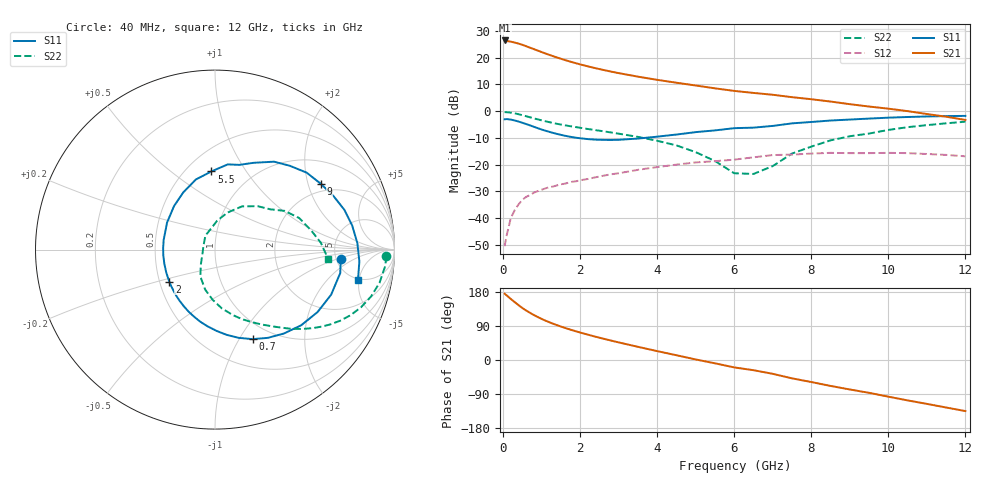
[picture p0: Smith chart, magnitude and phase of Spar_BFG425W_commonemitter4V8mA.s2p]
! Filename: 48bfg425.001
! BFG425W Field C1
! V1=8.298E-001V,V2=4.000E+000V, I1=8.674E-005A, I2=7.990E-003A
# GHz  S  MA  R 50
!  S11  S21  S12  S22
!Freq(GHz)  Mag  Ang  Mag  Ang  Mag  Ang  Mag  Ang
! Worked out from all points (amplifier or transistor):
!   44 points, 40 MHz to 12 GHz, reference 50 ohm
!   highest |S21| = 26.4 dB at 40 MHz (marker M1)
!   |S21| within 3 dB of that: start of sweep to 755.8 MHz
!   unconditionally stable (mu >= 1): 2.059 GHz to end of sweep
!   at 700 MHz: K = 0.48, MSG = 27.5 dB, |S12| = -31.4 dB
!   at 2.4 GHz: K = 1.08, MAG = 18.7 dB, |S12| = -24.7 dB
!   at 12 GHz: K = 1.42, MAG = 2.9 dB, |S12| = -16.9 dB
!   S11 on the Smith chart (normalised r, x): 40 MHz: 5.48, -1.17; 700 MHz: 0.81, -1.14; 2 GHz: 0.56, -0.22; 5.5 GHz: 0.66, +0.71; 9 GHz: 1.72, +2.43; 12 GHz: 4.87, -4.82
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0.04  0.703 -4.4  20.87 174.9  0.003 46.5  0.956 -2.2
0.2  0.694 -21.3  19.82 161.1  0.01 71.4  0.935 -11.4
0.3  0.669 -31.4  19.08 152.9  0.014 68.8  0.908 -16.7
0.4  0.639 -41.3  18.23 144.9  0.018 65.4  0.875 -21.5
0.5  0.605 -50.6  17.31 137.2  0.022 61.7  0.839 -25.8
0.6  0.573 -59.1  16.28 130.5  0.025 58.9  0.802 -29.6
0.7  0.541 -67.2  15.3 124.5  0.027 56.0  0.766 -32.9
0.9  0.48 -82.1  13.5 113.4  0.032 51.9  0.701 -38.6
1.2  0.41 -101.6  11.23 99.6  0.038 47.5  0.622 -45.2
1.4  0.375 -113.3  10.03 91.9  0.041 45.5  0.579 -48.9
1.6  0.347 -124.5  9.024 84.9  0.044 43.9  0.544 -52.2
2  0.311 -145.1  7.463 72.5  0.051 41.0  0.488 -58.5
2.2  0.3 -154.9  6.856 66.9  0.054 39.6  0.463 -61.7
3  0.291 169.5  5.123 46.5  0.069 33.3  0.379 -74.6
3.5  0.307 150.3  4.401 34.8  0.08 28.2  0.33 -83.3
4.5  0.365 118.8  3.388 12.6  0.1 16.1  0.229 -103.9
5.5  0.436 92.6  2.662 -8.8  0.116 2.1  0.117 -132.7
6.5  0.491 74.1  2.185 -26.9  0.137 -8.4  0.067 167.2
8.5  0.667 40.0  1.509 -68.4  0.166 -45.0  0.284 58.0
9  0.695 31.7  1.347 -77.8  0.164 -53.3  0.339 45.5
10.5  0.776 10.0  0.999 -106.6  0.164 -80.6  0.501 20.6
12  0.814 -11.8  0.683 -134.7  0.143 -111.4  0.634 -4.9
